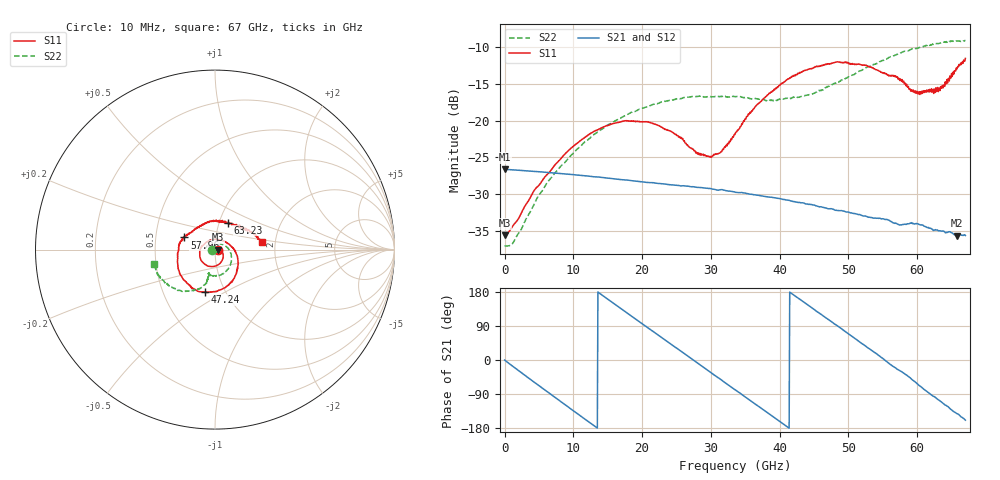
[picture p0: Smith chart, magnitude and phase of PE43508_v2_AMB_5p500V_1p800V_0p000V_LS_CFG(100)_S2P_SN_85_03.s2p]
!Keysight Technologies,N5227A,US51270237,A.10.43.00
!Date: Wednesday, August 22, 2018 17:17:06
!Correction: S11(Full 2 Port(1,3))
!S31(Full 2 Port(1,3))
!S13(Full 2 Port(1,3))
!S33(Full 2 Port(1,3))
!S2P File: Measurements: S11, S31, S13, S33:
# Hz S  dB  R 50
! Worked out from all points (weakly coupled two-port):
!   801 points, 10 MHz to 67 GHz, reference 50 ohm
!   highest |S21| = -26.61 dB at 10 MHz (marker M1); lowest = -35.7 dB at 65.83 GHz (marker M2)
!   lowest |S11| = -35.6 dB at 93.74 MHz (marker M3), VSWR 1.03, Z = 51.7 + j0.0176 ohm
!   |S11| at or under -10 dB: start of sweep to end of sweep
!   |S22| runs from -37.1 to -9.1 dB; largest |S21 - S12| = 0.00027
!   S11 on the Smith chart (normalised r, x): 10 MHz: 1.03, -0.00; 47.24 GHz: 0.80, -0.40; 57.96 GHz: 0.70, +0.10; 63.23 GHz: 1.10, +0.34; 67 GHz: 1.70, +0.15
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1e7  -35.51 -1.2  -26.61 -0.2  -26.61 -0.2  -37.09 -179.5
9.37375e7  -35.59 0.6  -26.63 -1.4  -26.64 -1.4  -37.06 176.6
1.266062e9  -34.26 5.9  -26.71 -17.6  -26.71 -17.6  -36.59 138.6
5.955362e9  -27.59 -14.9  -27.03 -80.4  -27.03 -80.4  -28.83 58.7
1.123082e10  -22.56 -59.9  -27.47 -150.1  -27.48 -150.1  -23.32 10.7
1.74274e10  -20.05 -111.7  -28.06 129.2  -28.06 129.2  -19.35 -31.1
2.236791e10  -20.66 -155.6  -28.56 65.2  -28.55 65.2  -17.62 -58.2
2.580115e10  -22.49 166.7  -28.87 21.4  -28.86 21.3  -16.96 -73.7
2.973681e10  -24.90 95.6  -29.23 -29.7  -29.23 -29.7  -16.69 -87.9
3.132782e10  -24.38 62.7  -29.41 -49.9  -29.42 -49.9  -16.71 -93.0
3.3505e10  -21.89 23.6  -29.72 -78.6  -29.73 -78.6  -16.72 -98.7
3.643581e10  -18.12 -13.4  -30.10 -116.1  -30.11 -116.1  -17.00 -103.5
3.88642e10  -16.11 -35.8  -30.45 -147.2  -30.45 -147.1  -17.26 -104.1
4.472582e10  -12.89 -84.1  -31.44 137.0  -31.43 137.1  -16.37 -103.2
4.723795e10  -12.32 -103.3  -31.99 105.1  -31.97 105.1  -15.33 -103.8
5.234594e10  -12.43 -144.1  -32.98 38.6  -32.95 38.5  -12.91 -110.2
5.586291e10  -13.93 -179.4  -33.55 -8.8  -33.53 -9.1  -11.41 -120.7
5.795635e10  -14.70 158.3  -34.14 -33.8  -34.15 -33.9  -10.61 -127.8
6.004979e10  -16.02 122.3  -34.03 -63.2  -34.04 -63.6  -10.16 -135.8
6.323181e10  -15.58 64.4  -34.99 -106.9  -35.02 -107.5  -9.47 -149.5
6.582768e10  -12.76 24.1  -35.68 -141.9  -35.76 -142.1  -9.19 -160.1
6.7e10  -11.53 8.9  -35.64 -158.8  -35.71 -159.0  -9.12 -166.6
